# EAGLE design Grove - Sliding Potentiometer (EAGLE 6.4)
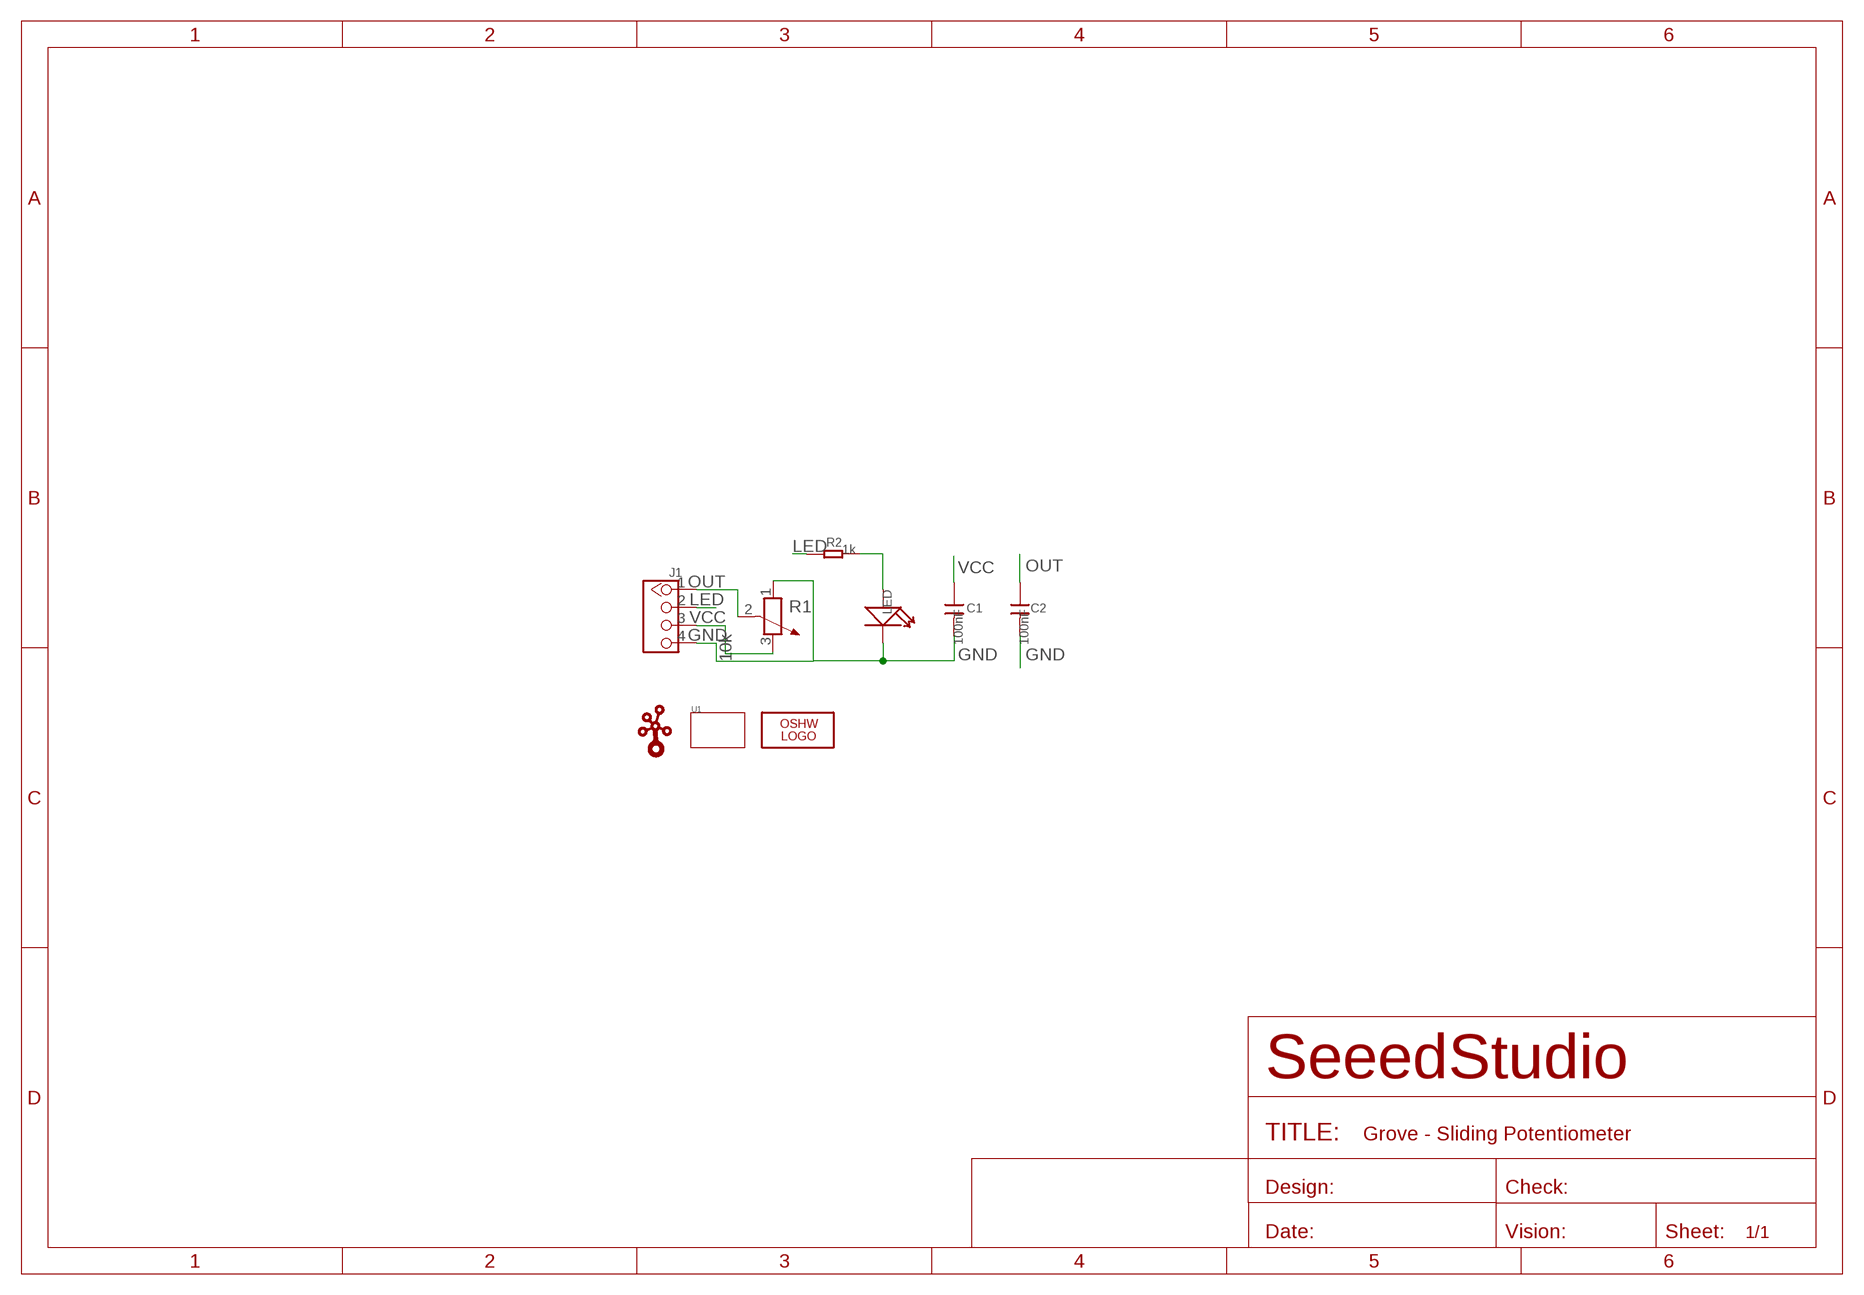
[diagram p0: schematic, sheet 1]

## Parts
C1  100nF  C-0805  [0805]
C2  100nF  C-0805  [0805]
J1  TWIG-4P-2.0-2.0  [4P-2.0]
LED  LED'0805'  [LED-0805]
LOGO1  LOGO-OSHW-FILLX0200-NT  [OSHW_FILLX200_NOTEXT]
R1  10k  R-POTENTIOMETER  [3P-SQUA-45.6X10X5.8H]
R2  1k  R-0805  [0805]
U1  TWIG'3U'  [3U-DIM-W/-DRILL]
U$1  LOGO-TWIG  [TWIGLOGO]

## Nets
GND: C1.2 C2.2 J1.4 LED.- R1.1
LED: J1.2 R2.1
N$5: LED.+ R2.2
OUT: C2.1 J1.1 R1.2
VCC: C1.1 J1.3 R1.3

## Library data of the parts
C1 C2 = Discrete:C*: Ceramic Capacitors
J1 = Connector:TWIG-4P-2.0
LED = Discrete:LED*
LOGO1 = Logo:LOGO-OSHW-FILL
R1 = Discrete:R-POTENTIOMETER*: Potentiometer
R2 = Discrete:R*
U1 = Module:TWIG
U$1 = Logo:LOGO-TWIG

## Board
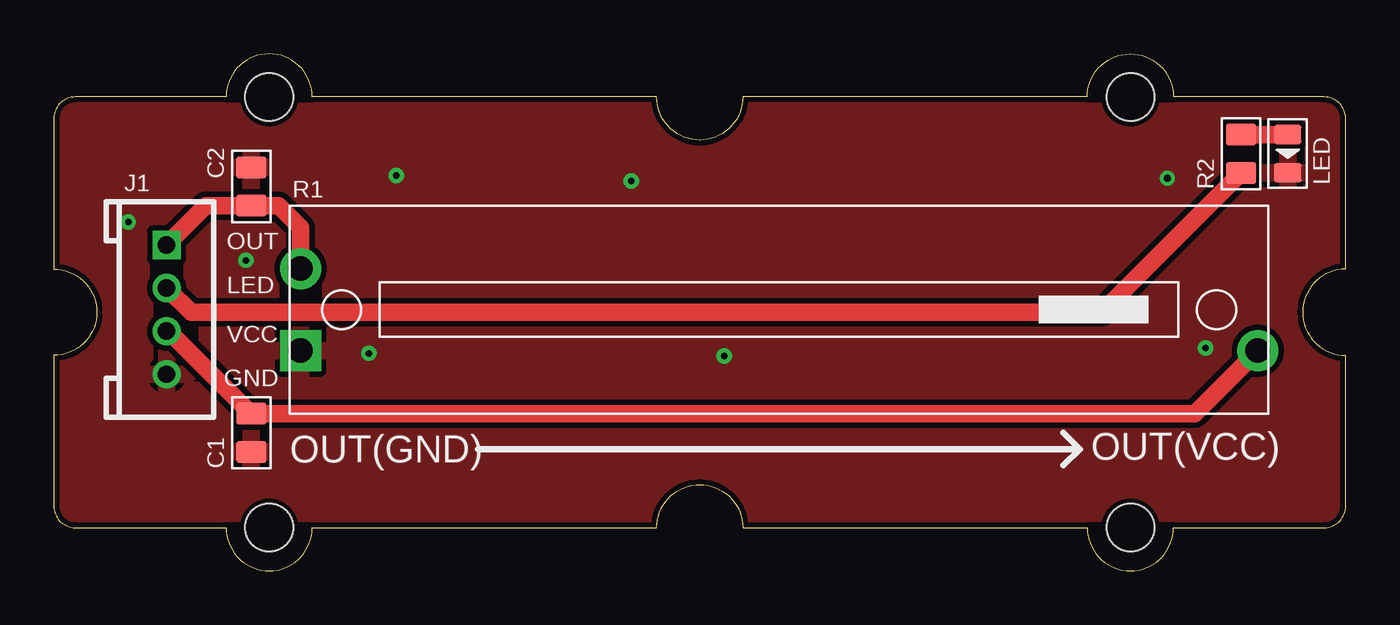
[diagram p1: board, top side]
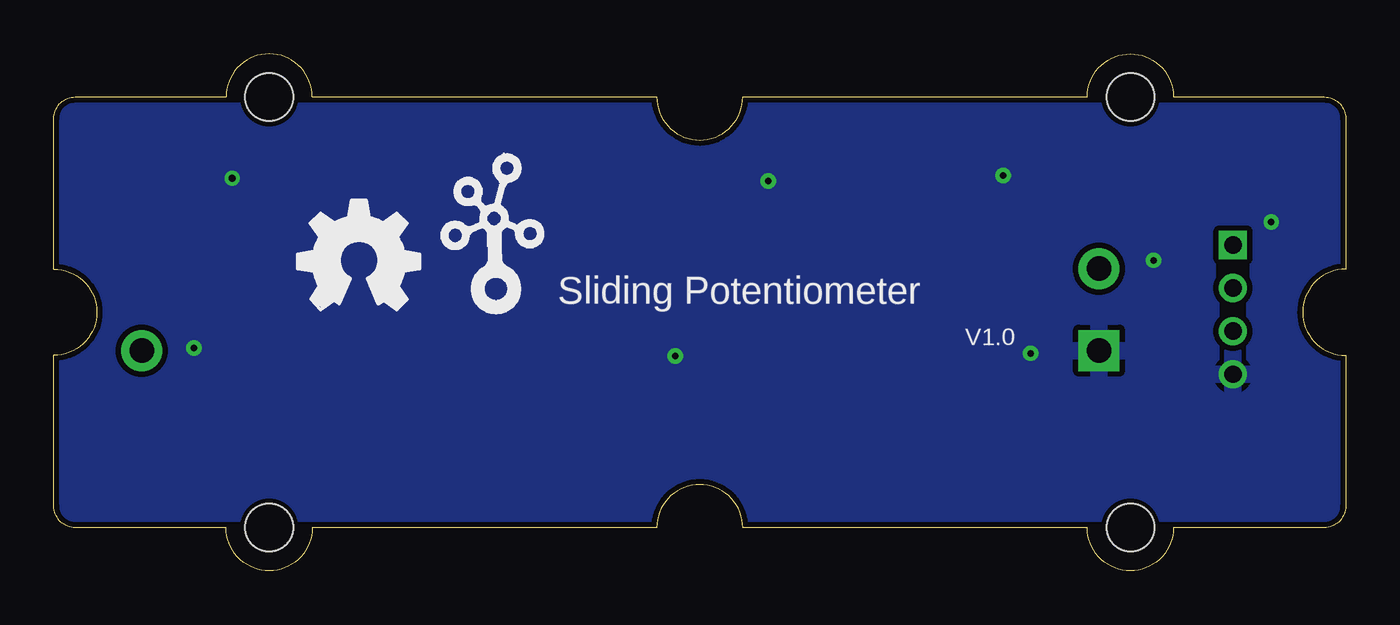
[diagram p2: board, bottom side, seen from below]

Size 60 x 24 mm. Coordinates in mm from the lower left corner, seen from the top.
Copper layers (1*16): Top 0.035mm / dielectric 1.5mm / Bottom 0.035mm
Design rules "default": minimum track width 6mil, minimum drill 12mil, track to track 6mil, track to pad 6mil, pad to pad 6mil, via to via 6mil, smd to smd 6mil, copper to edge 10mil, drill to drill 10mil, minimum pad ring 10mil, minimum via ring 8mil, stop-mask expansion 2mil, vias tented up to drill 100mil, thermal gap 10mil

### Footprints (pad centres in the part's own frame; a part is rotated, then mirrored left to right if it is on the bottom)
0805 = smd 1.016 x 1.397: 1 -0.889,0; 2 0.889,0
4P-2.0 = drill 0.8 pad 1.27 square: 1 -3,0 | drill 0.8 pad 1.27: 2 -1,0; 3 1,0; 4 3,0
LED-0805 = smd 0.889 x 1.27: + -0.889,0; - 0.889,0
3P-SQUA-45.6X10X5.8H = drill 1.143 pad 1.905 square: 1 -22.225,-1.905 | drill 1.143 pad 1.905: 2 -22.225,1.905; 3 22.225,-1.905
3U-DIM-W/-DRILL = hole 2.2: -20,10; -20,-10; 20,10; 20,-10

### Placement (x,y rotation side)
C1  9.17,6.41 270 top
C2  9.17,17.84 90 top
J1  5.23,12.13 270 top
LED  57.3,19.37 270 top
LOGO1  48.67,12.13 0 bottom
R1  33.68,12.13 0 top
R2  55.15,19.37 90 top
U1  30,12 0 top
U$1  39.52,12.89 0 bottom

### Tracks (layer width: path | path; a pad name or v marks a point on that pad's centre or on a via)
GND  (via drill 0.3 pad 0.64)
  other vias: 51.72,18.22 53.5,10.35 31.14,9.97 26.83,18.1 15.9,18.35 14.63,10.1 3.46,16.19 8.92,14.41
  pour Bottom (isolate 0.254): -3.15,25.08 -3.15,-2.86 62.89,-2.86 62.89,-1.59 62.89,26.35 -3.15,26.35
  pour Top (isolate 0.254): -0.61,-1.59 61.62,-1.59 61.62,25.08 -1.88,25.08 -1.88,-1.59
LED
  Top 0.813: J1.2 5.25,13.13 6.38,12 48.67,12 R2.1
N$5
  Top 0.813: R2.2 LED.+
OUT
  Top 0.813: R1.2 11.46,15.94 10.44,16.95 C2.1 7.06,16.95 J1.1
VCC
  Top 0.813: J1.3 5.35,11.13 C1.1 52.99,7.3 R1.3

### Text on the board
tPlace: OUT(VCC) | OUT(GND)
bPlace: Sliding Potentiometer | V1.0
tNames: OUT | LED | VCC | GND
